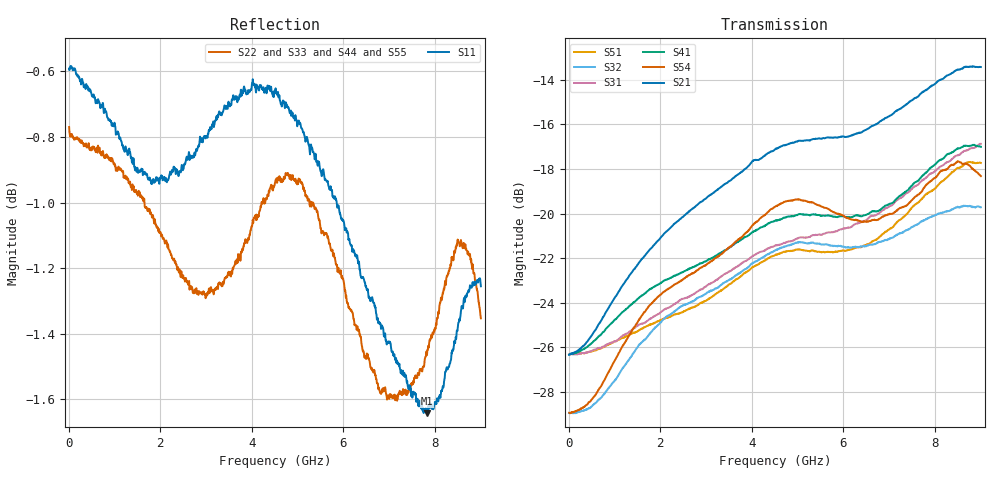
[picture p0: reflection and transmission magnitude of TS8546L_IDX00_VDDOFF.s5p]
# GHz S DB R 50
! CMT, SN0916, 25263762, 26.7.0
! Date: 16.07.2026 08:15:16
! Data: Format
! Freq S1.1:dB/Ang S1.2:dB/Ang S1.3:dB/Ang S1.4:dB/Ang S1.5:dB/Ang
!  S2.1:dB/Ang S2.2:dB/Ang S2.3:dB/Ang S2.4:dB/Ang S2.5:dB/Ang
!  S3.1:dB/Ang S3.2:dB/Ang S3.3:dB/Ang S3.4:dB/Ang S3.5:dB/Ang
!  S4.1:dB/Ang S4.2:dB/Ang S4.3:dB/Ang S4.4:dB/Ang S4.5:dB/Ang
!  S5.1:dB/Ang S5.2:dB/Ang S5.3:dB/Ang S5.4:dB/Ang S5.5:dB/Ang
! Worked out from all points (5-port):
!   2001 points, 10 MHz to 9 GHz, reference 50 ohm
!   strongest paths, dB at 10 MHz, 2.257 GHz, 4.505 GHz, 6.753 GHz, 9 GHz:
!     S21: -26.3, -20.6, -17.1, -15.9, -13.4
!     S54: -28.9, -23.3, -19.7, -20.3, -18.3
!     S41: -26.3, -22.8, -20.3, -19.9, -17.0
!     S31: -26.3, -24.1, -21.4, -20.0, -16.9
!     S32: -28.9, -24.5, -21.7, -21.3, -19.7
!     S51: -26.3, -24.6, -21.9, -21.1, -17.7
!   lowest |S11| = -1.6 dB at 7.822 GHz (marker M1), VSWR 10.61, Z = 13.9 + j68.8 ohm
!   |S11| at or under -10 dB: nowhere
